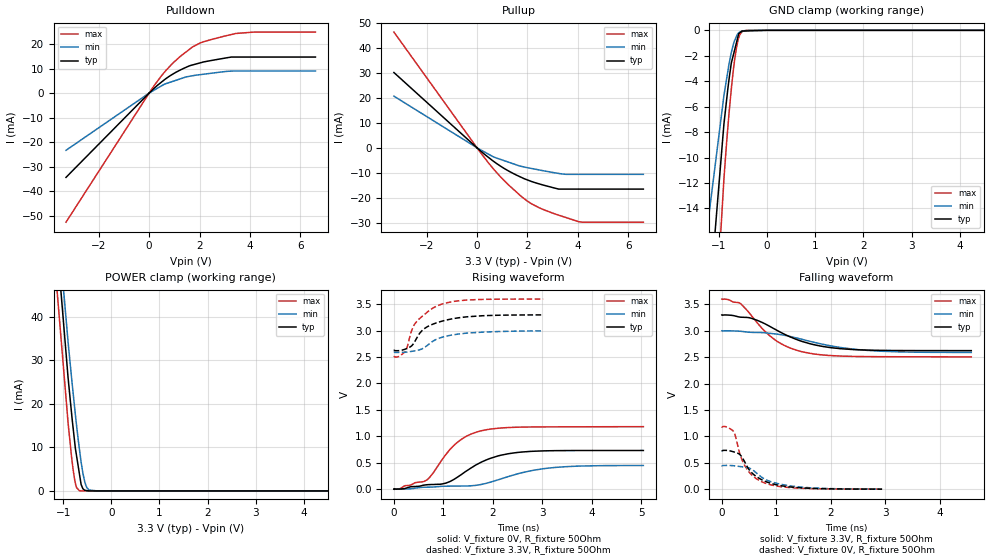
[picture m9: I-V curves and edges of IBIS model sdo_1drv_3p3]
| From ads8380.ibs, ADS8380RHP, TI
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|   sdo_1drv_3p3 Model
[Model]   sdo_1drv_3p3
Model_type   3-state
Polarity   Non-Inverting
Vmeas = 1.65
Vref = 1.65
Cref = 10pF
Rref = 50
|   typ   min   max
|   (nom PVT)   (fast PVT)   (slow PVT)
|C_comp from frequency sweep method (F=40MHz)
C_comp   5.648e-12   5.537e-12   5.708e-12
|ON state : BUFFER OUTPUT TURNED HIGH
|C_comp   5.487e-12   5.390e-12   5.564e-12
|OFF state: BUFFER IN HIGH IMPEDANCE
|C_comp   5.648e-12   5.537e-12   5.708e-12
|C_comp from LC tank measurement(L=1nH)
|Resonant Frequency(Hz)   3.970e+09   4.000e+09   3.910e+09
|C_comp   1.609e-12   1.585e-12   1.659e-12
|ON state : BUFFER OUTPUT TURNED HIGH
|Resonant Frequency(Hz)   3.970e+09   4.000e+09   3.910e+09
|C_comp   1.609e-12   1.585e-12   1.659e-12
|OFF state: BUFFER IN HIGH IMPEDANCE
|Resonant Frequency(Hz)   3.970e+09   3.990e+09   3.910e+09
|C_comp   1.609e-12   1.593e-12   1.659e-12
| Where nom  PVT is Nominal Process, 3.3V, 35C
|   Fast PVT is Strong Process,  3.6V, -40C
|   Slow PVT is Weak Process,   3V, 95C
[Voltage Range]   3.3   3   3.6
|Ambient Temperature   25   85   -40
|Junction Temperature
[Temperature Range]   35   95   -40
[Pullup Reference]   3.3   3   3.6
[Pulldown Reference]   0   0   0
[Power Clamp Reference]   3.3   3   3.6
[GND Clamp Reference]   0   0   0
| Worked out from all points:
|   slope of the pulldown table from 0 to 0.495 V, typ, clamps not added: 110 ohm
|   slope of the pullup table from 0 to 0.495 V, typ, clamps not added: 119 ohm
|   GND clamp passes 1 mA (typ) near -0.64 V on its own axis
|   POWER clamp passes 1 mA (typ) near -0.61 V on its own axis
|   falling waveform, V_fixture 3.3V, R_fixture 50Ohm: 20-80 % time 877ps typ, 1.14ns min, 676ps max; typ from 3.3 V to 2.62 V
|   rising waveform, V_fixture 0V, R_fixture 50Ohm: 20-80 % time 820ps typ, 1.06ns min, 635ps max; typ from 0 V to 0.732 V
|   rising waveform, V_fixture 3.3V, R_fixture 50Ohm: 20-80 % time 512ps typ, 562ps min, 435ps max; typ from 2.62 V to 3.3 V
|   falling waveform, V_fixture 0V, R_fixture 50Ohm: 20-80 % time 418ps typ, 527ps min, 318ps max; typ from 0.735 V to 0.003 V
[Pulldown]
|   Voltage   I(typ)   I(min)   I(max)
-3.3V     -34.29mA   -23.28mA   -52.53mA
208.8mV   2.055mA    1.263mA    3.19mA
633mV     5.65mA     3.722mA    8.819mA
939.6mV   7.745mA    4.778mA    12.19mA
1.464V    10.48mA    6.584mA    16.74mA
1.706V    11.41mA    7.025mA    18.66mA
2.203V    12.76mA    7.742mA    21.03mA
3.267V    14.67mA    8.959mA    23.84mA
3.449V    14.67mA    8.988mA    24.27mA
4.162V    14.67mA    8.995mA    24.82mA
6.6V      14.67mA    8.995mA    24.82mA
[GND Clamp]
|   Voltage   I(typ)   I(min)   I(max)
-3.3V     -300mA     -183.9mA   -660.5mA
-1.573V   -38.55mA   -27.45mA   -59mA
-1.224V   -22.44mA   -14.97mA   -32.48mA
-897.6mV  -7.374mA   -5.135mA   -11.71mA
-842.4mV  -5.499mA   -3.836mA   -8.853mA
-792mV    -3.869mA   -2.653mA   -6.546mA
-745.8mV  -2.607mA   -1.779mA   -4.695mA
-687.6mV  -1.73mA    -926.9uA   -2.685mA
-640.8mV  -1.025mA   -506uA     -1.451mA
-601.2mV  -429uA     -239.4uA   -723uA
-519mV    -57.29uA   -42.94uA   -108.9uA
6.6V      0A         0A         0A
[Pullup]
|   Voltage   I(typ)   I(min)   I(max)
-3.3V     30.09mA    20.64mA    46.24mA
18mV      -159.1uA   -110.6uA   -251.5uA
478.8mV   -4.019mA   -2.667mA   -6.334mA
702mV     -5.726mA   -3.821mA   -9.019mA
1.228V    -9.118mA   -5.644mA   -14.59mA
1.861V    -12.28mA   -7.639mA   -20.25mA
2.167V    -13.46mA   -8.254mA   -22.38mA
2.473V    -14.42mA   -8.845mA   -23.97mA
3.241V    -16.48mA   -10.22mA   -26.89mA
4.032V    -16.48mA   -10.59mA   -29.5mA
6.6V      -16.48mA   -10.59mA   -29.69mA
[POWER Clamp]
|   Voltage   I(typ)   I(min)   I(max)
-3.3V     597.5mA    489.1mA    865.1mA
-1.156V   60.55mA    67.18mA    49.96mA
-897.6mV  26.03mA    34.25mA    15.65mA
-824.4mV  17.75mA    25.92mA    7.74mA
-766.8mV  11.86mA    19.74mA    2.964mA
-720mV    7.952mA    14.91mA    731.1uA
-662.4mV  3.944mA    9.643mA    56.93uA
-627mV    1.481mA    6.651mA    11.79uA
-549mV    129uA      1.968mA    6.895uA
-510mV    73.36uA    791.2uA    4.446uA
-462mV    4.874uA    205uA      1.433uA
6.6V      0A         0A         0A
[Ramp]
R_load = 50
|   typ   min   max
dV/dt_r   0.440795/8.24418e-10   0.269812/1.06483e-09   0.71098/6.36047e-10
dV/dt_f   0.406398/8.81323e-10   0.246943/1.13833e-09   0.657151/6.77744e-10
[Falling Waveform]
V_fixture = 3.3V
V_fixture_min = 3V
V_fixture_max = 3.6V
R_fixture = 50Ohm
|   Time   V(typ)   V(min)   V(max)
0s        3.3V       3V         3.6V
344ps     3.258V     2.991V     3.516V
546ps     3.236V     2.97V      3.285V
754ps     3.152V     2.965V     3.03V
946ps     3.046V     2.945V     2.852V
1.192ns   2.914V     2.907V     2.701V
1.474ns   2.799V     2.838V     2.603V
2.004ns   2.681V     2.714V     2.531V
2.67ns    2.635V     2.63V      2.512V
4.58ns    2.625V     2.59V      2.507V
[Rising Waveform]
V_fixture = 0V
V_fixture_min = 0V
V_fixture_max = 0V
R_fixture = 50Ohm
|   Time   V(typ)   V(min)   V(max)
0s        5.07nV     10.05nV    4.701nV
664ps     82.77mV    36.6mV     172.5mV
778ps     87.41mV    38.68mV    287.4mV
976ps     98.07mV    53.36mV    562.1mV
1.214ns   184.9mV    57mV       829.9mV
1.444ns   330.5mV    58.98mV    990.9mV
1.744ns   500.8mV    85mV       1.1V
2.312ns   670mV      238.4mV    1.166V
3.084ns   725.4mV    393.8mV    1.178V
5.038ns   731.6mV    447.9mV    1.182V
[Rising Waveform]
V_fixture = 3.3V
V_fixture_min = 3V
V_fixture_max = 3.6V
R_fixture = 50Ohm
|   Time   V(typ)   V(min)   V(max)
0s        2.623V     2.588V     2.505V
106ps     2.622V     2.587V     2.513V
234ps     2.651V     2.592V     2.611V
268ps     2.664V     2.595V     2.689V
364ps     2.717V     2.608V     3.017V
446ps     2.833V     2.621V     3.158V
608ps     3.033V     2.675V     3.298V
904ps     3.161V     2.853V     3.48V
1.496ns   3.263V     2.955V     3.58V
3.014ns   3.298V     2.996V     3.597V
[Falling Waveform]
V_fixture = 0V
V_fixture_min = 0V
V_fixture_max = 0V
R_fixture = 50Ohm
|   Time   V(typ)   V(min)   V(max)
0s        734.8mV    450.1mV    1.185V
206ps     712.3mV    447.6mV    1.107V
254ps     698.2mV    442.1mV    990.4mV
350ps     637.6mV    429.5mV    612.4mV
458ps     443.4mV    414.1mV    386.2mV
578ps     286.8mV    357.4mV    244.4mV
778ps     159.3mV    199.2mV    123.7mV
1.018ns   81.91mV    111mV      60.23mV
1.422ns   30.59mV    44.89mV    21.3mV
2.942ns   3.243mV    3.091mV    3.915mV
